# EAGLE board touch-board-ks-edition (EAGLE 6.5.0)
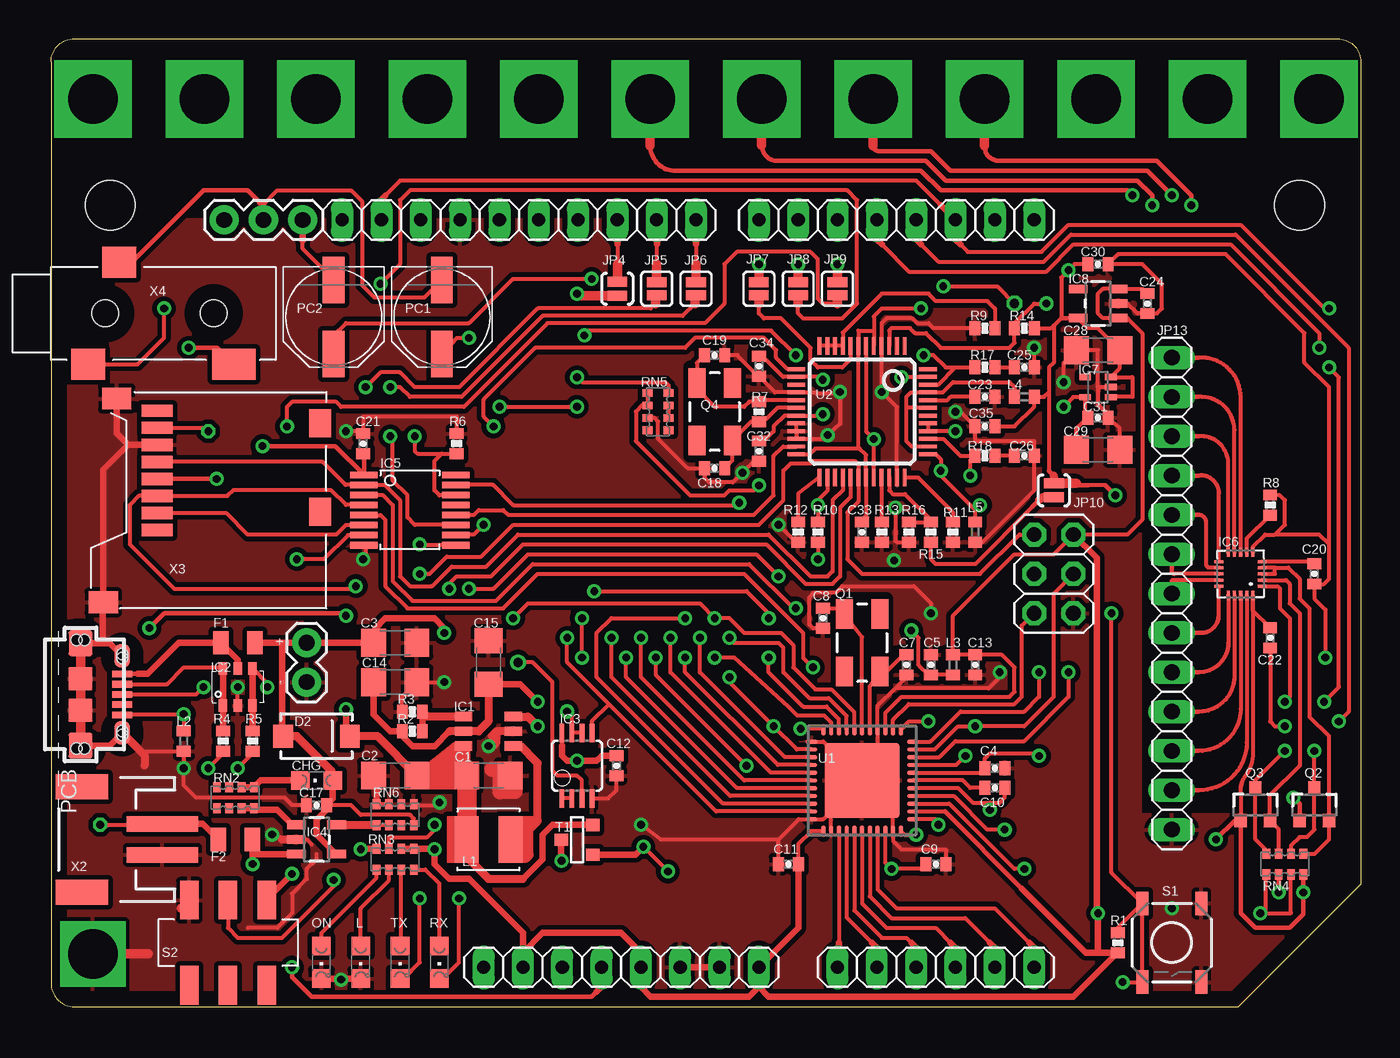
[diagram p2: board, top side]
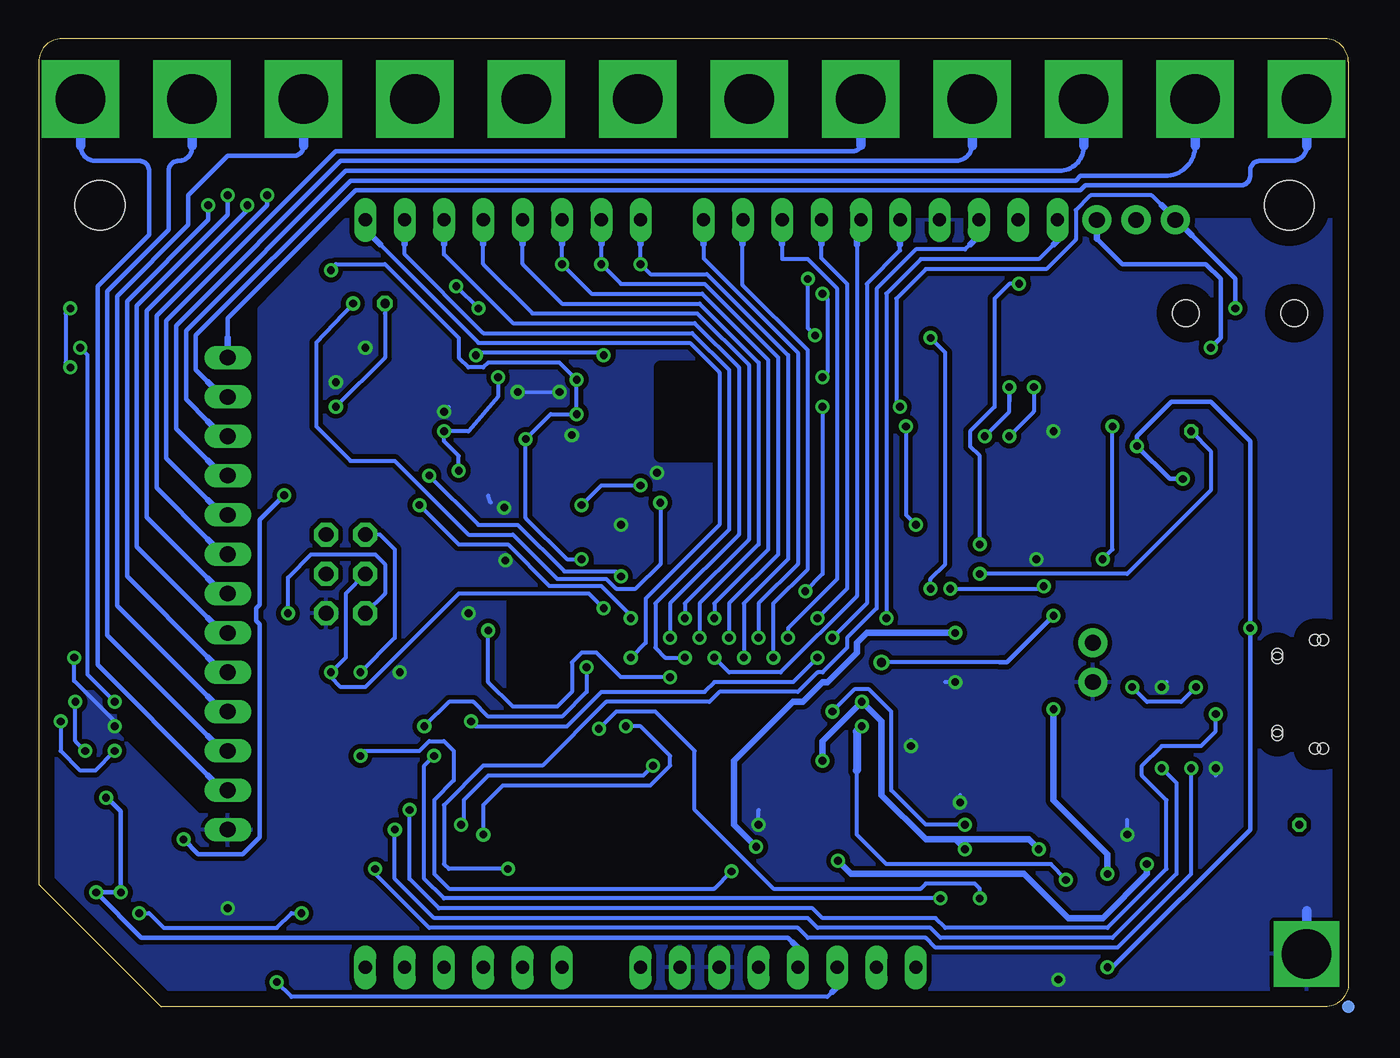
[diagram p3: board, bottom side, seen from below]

Size 84.6 x 62.5 mm. Coordinates in mm from the lower left corner, seen from the top.
Outline: 0,61 0,1.5 arc90 1.5,0 76.7,0 84.6,7.9 84.6,61 arc90 83.1,62.5 1.5,62.5 arc90 0,61
Copper layers (1*16): Top 0.035mm / dielectric 1.5mm / Bottom 0.035mm
Design rules "default *": minimum track width 10mil, minimum drill 20mil, track to track 8mil, track to pad 8mil, pad to pad 8mil, via to via 8mil, smd to smd 8mil, copper to edge 40mil, drill to drill 8mil, minimum pad ring 10mil, minimum via ring 8mil, stop-mask expansion 1.25mil, vias tented up to drill 0mil, thermal gap 10mil
Net classes: 1 power: width 0.254 mm, drill 0.61 mm, clearance 0.254 mm; 2 gnd: width 0.254 mm, drill 0.61 mm, clearance 0.254 mm; 3 usbvcc: width 0.254 mm, drill 0.61 mm, clearance 0.254 mm; 4 aref: width 0.254 mm, drill 0.61 mm, clearance 0.254 mm
Holes 3.2 mm at 80.64,51.75 3.81,51.75
tRestrict: area 41.3,35.6 to 44.5,41.3; area 50.8,20.6 to 54,26.4; area 27.6,9.4 to 28.9,12.2
bRestrict: area 41.3,35.6 to 44.5,41.3; area 50.8,20.6 to 54,26.4

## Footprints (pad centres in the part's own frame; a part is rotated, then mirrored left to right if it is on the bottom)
1206 = smd 1.6 x 1.8: 1 -1.4,0; 2 1.4,0
0402-CAP = smd 0.7 x 0.9: 1 -0.65,0; 2 0.65,0
CHIPLED_0805 = smd 1.2 x 1.2: A 0,-1.05; C 0,1.05
SMA-DIODE = smd 1.27 x 1.47: A -2.15,0; C 2.15,0
0805 = smd 1 x 1.5: 1 -1.1,0; 2 1.1,0
6-LEAD-SOT23 = smd 0.6 x 1.1: 1 -0.95,-1.6; 2 0,-1.6; 3 0.95,-1.6; 4 0.95,1.6; 5 0,1.6; 6 -0.95,1.6
SOT457 = smd 0.8 x 0.55: 1 -1.2,0.95; 2 -1.2,0; 3 -1.2,-0.95; 4 1.2,-0.95; 5 1.2,0; 6 1.2,0.95
MSOP08 = smd 0.3 x 1.2: 1 -0.976,-2.113; 2 -0.326,-2.113; 3 0.324,-2.113; 4 0.974,-2.113; 5 0.974,2.112; 6 0.324,2.112; 7 -0.326,2.112; 8 -0.976,2.112
SOT23-5 = smd 0.55 x 1.2: 1 -0.95,-1.3; 2 0,-1.3; 3 0.95,-1.3; 4 0.95,1.3; 5 -0.95,1.3
TSSOP-16 = smd 0.42 x 1.78: 1 -2.275,-2.97; 2 -1.625,-2.97; 3 -0.975,-2.97; 4 -0.325,-2.97; 5 0.325,-2.97; 6 0.975,-2.97; 7 1.625,-2.97; 8 2.275,-2.97; 9 2.275,2.97; 10 1.625,2.97; 11 0.975,2.97; 12 0.325,2.97; 13 -0.325,2.97; 14 -0.975,2.97; 15 -1.625,2.97; 16 -2.275,2.97
QFN-20-0.4MM = smd 0.6 x 0.2: 1 -1.4,0.8; 2 -1.4,0.4; 3 -1.4,0; 4 -1.4,-0.4; 5 -1.4,-0.8; 11 1.4,-0.8; 12 1.4,-0.4; 13 1.4,0; 14 1.4,0.4; 15 1.4,0.8 | smd 0.2 x 0.6: 6 -0.8,-1.4; 7 -0.4,-1.4; 8 0,-1.4; 9 0.4,-1.4; 10 0.8,-1.4; 16 0.8,1.4; 17 0.4,1.4; 18 0,1.4; 19 -0.4,1.4; 20 -0.8,1.4
SC70 = smd 0.4 x 0.75: 1 -0.65,-0.825; 2 0,-0.825; 3 0.65,-0.825; 4 0.65,0.825; 5 -0.65,0.825
2X03 = drill 0.95 pad 1.55 octagon: 1 -2.54,-1.27; 2 -2.54,1.27; 3 0,-1.27; 4 0,1.27; 5 2.54,-1.27; 6 2.54,1.27
1X08 = drill 0.85 pad 1.422 long: 1 -8.89,0; 2 -6.35,0; 3 -3.81,0; 4 -1.27,0; 5 1.27,0; 6 3.81,0; 7 6.35,0; 8 8.89,0
1X06 = drill 0.85 pad 1.422 long: 1 -6.35,0; 2 -3.81,0; 3 -1.27,0; 4 1.27,0; 5 3.81,0; 6 6.35,0
1X02 = drill 1.016 pad 1.88: 1 0,0; 2 2.54,0
1X10 = drill 0.85 pad 1.422 long: 1 -11.43,0; 2 -8.89,0; 3 -6.35,0; 4 -3.81,0; 5 -1.27,0; 6 1.27,0; 7 3.81,0; 8 6.35,0; 9 8.89,0; 10 11.43,0
SJ_2S-NO = smd 0.635 x 1.27: 1 -0.45,0; 2 0.45,0
SJ_2S = smd 0.635 x 1.27: 1 -0.412,0; 2 0.412,0
1X03 = drill 1.016 pad 1.88: 1 0,0; 2 2.54,0; 3 5.08,0
1X13 = drill 1.016 long: 1 -15.24,0; 2 -12.7,0; 3 -10.16,0; 4 -7.62,0; 5 -5.08,0; 6 -2.54,0; 7 0,0; 8 2.54,0; 9 5.08,0; 10 7.62,0; 11 10.16,0; 12 12.7,0; 13 15.24,0
LQH44PN100MP0L = smd 1.55 x 3: 1 -1.425,0; 2 1.425,0
0402 = smd 0.7 x 0.9: 1 -0.65,0; 2 0.65,0
TP-SP = smd 0.8 x 0.8 bottom: X 0,0
PANASONIC_D = smd 3 x 1.4: + 2.4,0; - -2.4,0
CRYSTAL-SMD-5X3 = smd 1.9 x 1.1: 1 -1.85,-1.15; 2 1.85,-1.15; 3 1.85,1.15; 4 -1.85,1.15
SOT23-3 = smd 0.8 x 0.9: 1 -0.95,-1; 2 0.95,-1; 3 0,1.1
0402-RES = smd 0.7 x 0.9: 1 -0.65,0; 2 0.65,0
CAY16 = smd 0.5 x 0.65: 1 -1.2,-0.675; 2 -0.4,-0.675; 3 0.4,-0.675; 4 1.2,-0.675; 5 1.2,0.675; 6 0.4,0.675; 7 -0.4,0.675; 8 -1.2,0.675
TACTILE_SWITCH_SMD@1 = smd 1.524 x 0.762: 1 -2.54,1.905; 2 2.54,1.905; 3 -2.54,-1.905; 4 2.54,-1.905
JS202011SCQN = smd 1.2 x 2.5: 1 -2.5,-2.75; 2 0,-2.75; 3 2.5,-2.75; 4 -2.5,2.75; 5 0,2.75; 6 2.5,2.75
SOT-23 = smd 0.787 x 0.889: 1 0.025,-1.016; 2 -0.94,1.016; 3 0.991,1.016
QFN44ML7X7 = smd 0.75 x 0.275: 1 -3.275,2.5; 2 -3.275,2; 3 -3.275,1.5; 4 -3.275,1; 5 -3.275,0.5; 6 -3.275,0; 7 -3.275,-0.5; 8 -3.275,-1; 9 -3.275,-1.5; 10 -3.275,-2; 11 -3.275,-2.5; 23 3.275,-2.5; 24 3.275,-2; 25 3.275,-1.5; 26 3.275,-1; 27 3.275,-0.5; 28 3.275,0; 29 3.275,0.5; 30 3.275,1; 31 3.275,1.5; 32 3.275,2; 33 3.275,2.5 | smd 0.275 x 0.75: 12 -2.5,-3.275; 13 -2,-3.275; 14 -1.5,-3.275; 15 -1,-3.275; 16 -0.5,-3.275; 17 0,-3.275; 18 0.5,-3.275; 19 1,-3.275; 20 1.5,-3.275; 21 2,-3.275; 22 2.5,-3.275; 34 2.5,3.275; 35 2,3.275; 36 1.5,3.275; 37 1,3.275; 38 0.5,3.275; 39 0,3.275; 40 -0.5,3.275; 41 -1,3.275; 42 -1.5,3.275; 43 -2,3.275; 44 -2.5,3.275 | smd 4.826 x 4.826: EXP 0,0
LQFP-48 = smd 0.254 x 1.143: 1 -2.75,-4.25; 2 -2.25,-4.25; 3 -1.75,-4.25; 4 -1.25,-4.25; 5 -0.75,-4.25; 6 -0.25,-4.25; 7 0.25,-4.25; 8 0.75,-4.25; 9 1.25,-4.25; 10 1.75,-4.25; 11 2.25,-4.25; 12 2.75,-4.25; 25 2.75,4.25; 26 2.25,4.25; 27 1.75,4.25; 28 1.25,4.25; 29 0.75,4.25; 30 0.25,4.25; 31 -0.25,4.25; 32 -0.75,4.25; 33 -1.25,4.25; 34 -1.75,4.25; 35 -2.25,4.25; 36 -2.75,4.25 | smd 1.143 x 0.254: 13 4.25,-2.75; 14 4.25,-2.25; 15 4.25,-1.75; 16 4.25,-1.25; 17 4.25,-0.75; 18 4.25,-0.25; 19 4.25,0.25; 20 4.25,0.75; 21 4.25,1.25; 22 4.25,1.75; 23 4.25,2.25; 24 4.25,2.75; 37 -4.25,2.75; 38 -4.25,2.25; 39 -4.25,1.75; 40 -4.25,1.25; 41 -4.25,0.75; 42 -4.25,0.25; 43 -4.25,-0.25; 44 -4.25,-0.75; 45 -4.25,-1.25; 46 -4.25,-1.75; 47 -4.25,-2.25; 48 -4.25,-2.75
EDGE-ELEC-LEFT = drill 3.2 pad 5 square: 1 0,0
EDGE-ELEC-RIGHT = drill 3.2 pad 5 square: 1 0,0
EDGE-GND = drill 3.2 pad 4 square: P$1 0,0
EDGE-ELEC = drill 3.2 pad 5 square: 1 0,0
CON2_USB_MICRO_B_AT = smd 0.406 x 1.346: P1 -1.321,2.692; P2 -0.66,2.692; P3 0,2.692; P4 0.66,2.692; P5 1.321,2.692 | smd 1.651 x 1.549: S1 -3.302,0; S2 3.302,0 | smd 1.524 x 1.016: S3 -2.489,2.692; S4 2.489,2.692 | smd 1.524 x 1.524: S5 -1.016,0; S6 1.016,0 | hole 0.7: -3.505,0.254; -3.505,-0.254; 3.505,0.254; 3.505,-0.254; -2.616,2.692; -2.362,2.692; 2.362,2.692; 2.616,2.692
JST-2-SMD = smd 1 x 4.6: 1 -1,-3.7; 2 1,-3.7 | smd 1.6 x 3.4: NC1 -3.4,1.5; NC2 3.4,1.5
MSDC-PP-02 = smd 0.8 x 2: 1 5.06,10.94; 2 6.16,10.94; 3 7.26,10.94; 4 8.36,10.94; 5 9.46,10.94; 6 10.56,10.94; 7 11.66,10.94; 8 12.76,10.94 | smd 1.8 x 1.4: CD1 6.25,0.4; CD2 11.95,0.4 | smd 1.4 x 1.9: S1 0.4,14.4; S2 13.55,13.54
3POLE-JACK = smd 2.2 x 2: 1 2.4,-3.3; 3 4.4,3.3 | smd 2.8 x 2: 2 11.8,-3.3 | hole 1.7: 3.5,0; 10.5,0

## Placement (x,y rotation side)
C1  10uF  [1206]  28.26,14.92 0 top
C2  10uF  [1206]  22.23,14.92 180 top
C3  10uF  [1206]  22.23,23.5 0 top
C4  0.1uF  [0402-CAP]  60.96,15.4 180 top
C5  1uF  [0402-CAP]  56.83,22.07 270 top
C7  22pF  [0402-CAP]  55.24,22.07 270 top
C8  22pF  [0402-CAP]  49.85,25.08 270 top
C9  0.1uF  [0402-CAP]  57.15,9.21 180 top
C10  1uF  [0402-CAP]  60.96,14.13 180 top
C11  0.1uF  [0402-CAP]  47.62,9.21 0 top
C12  0.1uF  [0402-CAP]  36.51,15.56 90 top
C13  0.1uF  [0402-CAP]  59.69,22.07 90 top
C14  10uF  [1206]  22.23,20.95 0 top
C15  10uF  [1206]  28.26,22.23 90 top
C17  1uF  [0402-CAP]  17.14,13.02 0 top
C18  22pF  [0402-CAP]  42.86,34.77 180 top
C19  22pF  [0402-CAP]  42.86,42.07 0 top
C20  0.1uF  [0402-CAP]  81.6,27.94 90 top
C21  0.1uF  [0402-CAP]  20.16,36.35 270 top
C22  0.1uF  [0402-CAP]  78.74,23.81 90 top
C23  1uF  [0402-CAP]  60.33,39.37 0 top
C24  1uF  [0402-CAP]  70.8,45.4 90 top
C25  0.01uF  [0402-CAP]  62.87,41.27 180 top
C26  0.01uF  [0402-CAP]  62.87,35.56 180 top
C28  10uF  [1206]  67.63,42.39 180 top
C29  10uF  [1206]  67.63,35.96 0 top
C30  0.1uF  [0402-CAP]  67.63,47.94 180 top
C31  0.1uF  [0402-CAP]  67.63,38.02 180 top
C32  0.1uF  [0402-CAP]  45.72,35.88 90 top
C33  0.1uF  [0402-CAP]  52.39,30.64 90 top
C34  0.1uF  [0402-CAP]  45.72,41.35 90 top
C35  0.1uF  [0402-CAP]  60.33,37.47 0 top
CHG  Yellow  [CHIPLED_0805]  17.14,14.61 90 top
D2  B340  [SMA-DIODE]  17.14,17.46 0 top
F1  500mA  [0805]  12.06,23.5 0 top
F2  1.1A  [0805]  11.91,10.79 0 top
IC1  MCP1640  [6-LEAD-SOT23]  28.26,17.78 90 top
IC2  ESD Diode  [SOT457]  12.06,20.64 90 top
IC3  LM358  [MSOP08]  33.97,15.56 0 top
IC4  MCP73831  [SOT23-5]  17.14,10.79 270 top
IC5  74HC4050  [TSSOP-16]  23.18,32.07 270 top
IC6  MPR121  [QFN-20-0.4MM]  76.83,27.94 180 top
IC7  1.8V  [SC70]  67.63,40.01 90 top
IC8  MIC5219  [SOT23-5]  67.63,45.4 90 top
ICSP  ICSP  [2X03]  64.77,27.94 270 top
J1  8x1F-H8.5  [1X08]  36.83,2.54 0 top
J2  6x1F-H8.5  [1X06]  57.15,2.54 0 top
J3  8x1F-H8.5  [1X08]  54.61,50.8 180 top
JP1  External  [1X02]  16.51,20.95 90 top
JP3  10x1F-H8.5  [1X10]  30.23,50.8 180 top
JP4  [SJ_2S-NO]  36.58,46.35 90 top
JP5  [SJ_2S]  39.12,46.35 90 top
JP6  [SJ_2S]  41.66,46.35 90 top
JP7  [SJ_2S]  45.72,46.35 90 top
JP8  [SJ_2S]  48.26,46.35 90 top
JP9  [SJ_2S]  50.8,46.35 90 top
JP10  [SJ_2S-NO]  64.77,33.34 90 top
JP11  External Speaker  [1X03]  11.18,50.8 0 top
JP13  Touch Electrodes  [1X13]  72.39,26.67 270 top
L  Red  [CHIPLED_0805]  20,2.86 180 top
L1  LQH44P  [LQH44PN100MP0L]  28.26,10.79 180 top
L2  Ferrite  [0402]  8.57,17.14 90 top
L3  [0402]  58.26,22.07 270 top
L4  Ferrite  [0402]  62.87,39.37 180 top
L5  Ferrite  [0402]  59.69,30.64 270 top
ON  Green  [CHIPLED_0805]  17.46,2.86 180 top
ORIGIN  TP_SP  [TP-SP]  0,0 0 top
PC1  220uF  [PANASONIC_D]  25.24,44.53 270 top
PC2  220uF  [PANASONIC_D]  18.26,44.53 270 top
Q1  16MHz  [CRYSTAL-SMD-5X3]  52.39,23.5 270 top
Q2  BSS138  [SOT23-3]  81.6,13.02 0 top
Q3  BSS138  [SOT23-3]  77.79,13.02 0 top
Q4  12.288MHz  [CRYSTAL-SMD-5X3]  42.86,38.42 270 top
R1  75k  [0402-RES]  68.9,4.13 90 top
R2  976K  [0402-RES]  23.34,17.78 180 top
R3  309K  [0402-RES]  23.34,19.05 180 top
R4  22R  [0402-RES]  11.11,17.14 270 top
R5  22R  [0402-RES]  13.02,17.14 270 top
R6  75k  [0402-RES]  26.19,36.35 90 top
R7  976k  [0402-RES]  45.72,38.42 90 top
R8  75k  [0402-RES]  78.74,32.38 90 top
R9  75k  [0402-RES]  60.33,43.81 180 top
R10  75k  [0402-RES]  48.26,30.64 270 top
R11  75k  [0402-RES]  58.26,30.64 270 top
R12  75k  [0402-RES]  49.53,30.64 90 top
R13  75k  [0402-RES]  53.66,30.64 270 top
R14  75k  [0402-RES]  62.87,43.81 180 top
R15  75k  [0402-RES]  55.4,30.64 270 top
R16  75k  [0402-RES]  56.83,30.64 90 top
R17  22R  [0402-RES]  60.33,41.27 0 top
R18  22R  [0402-RES]  60.33,35.56 0 top
RN2  1K  [CAY16]  11.91,13.49 180 top
RN3  1K  [CAY16]  22.23,9.53 180 top
RN4  1K  [CAY16]  79.69,9.21 180 top
RN5  10k  [CAY16]  39.21,38.42 270 top
RN6  10K  [CAY16]  22.23,12.38 0 top
RX  Yellow  [CHIPLED_0805]  25.08,2.86 180 top
S1  RESET  [TACTILE_SWITCH_SMD@1]  72.39,4.13 270 top
S2  DPDT  [JS202011SCQN]  11.43,4.13 0 top
T1  FDN340P  [SOT-23]  33.97,10.79 270 top
TX  Yellow  [CHIPLED_0805]  22.54,2.86 180 top
U1  ATMEGA32U4  [QFN44ML7X7]  52.39,14.61 180 top
U2  VS1053  [LQFP-48]  52.39,38.42 180 top
U$1  EDGE-ELEC-LEFT  [EDGE-ELEC-LEFT]  2.7,58.6 0 top
U$3  EDGE-ELEC-RIGHT  [EDGE-ELEC-RIGHT]  81.9,58.6 0 top
U$6  EDGE-GND  [EDGE-GND]  2.7,3.4 0 top
U$8  OSHW-LOGO  [OSHW-LOGO]  not placed on the board
U$17  EDGE-ELEC  [EDGE-ELEC]  74.7,58.6 0 top
U$18  EDGE-ELEC  [EDGE-ELEC]  67.5,58.6 0 top
U$22  EDGE-ELEC  [EDGE-ELEC]  60.3,58.6 0 top
U$24  EDGE-ELEC  [EDGE-ELEC]  53.1,58.6 0 top
U$26  EDGE-ELEC  [EDGE-ELEC]  45.9,58.6 0 top
U$27  EDGE-ELEC  [EDGE-ELEC]  38.7,58.6 0 top
U$28  EDGE-ELEC  [EDGE-ELEC]  31.5,58.6 0 top
U$29  EDGE-ELEC  [EDGE-ELEC]  24.3,58.6 0 top
U$30  EDGE-ELEC  [EDGE-ELEC]  17.1,58.6 0 top
U$31  EDGE-ELEC  [EDGE-ELEC]  9.9,58.6 0 top
X1  USB MICRO  [CON2_USB_MICRO_B_AT]  1.91,20.16 270 top
X2  Batt  [JST-2-SMD]  3.49,10.79 90 top
X3  MICRO-SD  [MSDC-PP-02]  17.78,25.72 90 top
X4  [3POLE-JACK]  0,44.77 0 top

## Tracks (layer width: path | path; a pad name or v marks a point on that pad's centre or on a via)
1.8V  (via drill 0.5, 0.6)
  Top 0.254: C29.1 66.23,37.35 C31.2 66.8,38.27 IC7.5 66.03,39.35 v65.41,38.73 | U2.24 49,35.67 49.37,36.04 52.23,36.04 | C33.2 52.39,31.43 52.64,31.68 U2.31 52.64,35.63 52.23,36.04 | v56.2,45.09 53.66,45.09 53.14,44.56 U2.5 53.14,43.66 52.14,43.66 U2.7 52.14,36.13 52.23,36.04 | v57.63,46.51 61.12,46.51 v62.23,45.4
  Bottom 0.254: v57.63,46.51 v56.2,45.09 | v65.41,38.73 62.23,41.91 62.23,44.77 v62.23,45.4
3.3V  (via drill 0.5, 0.6)
  Top 0.254: RN4.8 80.96,8.46 | Q3.1 76.83,12.33 | 76.83,12.34 Q3.1 | C22.2 77.64,25.57 IC6.20 77.64,16.36 arc-37 77.15,14.92 arc42 76.83,13.81 76.83,12.34 | U2.6 52.64,37.15 v53.14,36.65 U2.32 | IC7.1 68.47,39.37 69.85,39.37 69.85,40.64 69.83,40.66 IC7.3 69.03,41.23 C28.1 69.03,42.41 67.63,43.81 66.97,43.81 IC8.5 | v49.85,38.26 49.85,38.17 U2.19 47.38,38.17 46.67,37.47 46.67,37.15 46.05,36.53 C32.2 | v49.85,40.48 49.85,40.67 U2.14 47.28,40.67 45.95,42 C34.2 | R12.1 v49.53,28.89 | 76.83,12.34 76.83,12.33 | 20.21,35.66 C21.2 | 65.25,44.45 | 65.25,44.45 IC8.5 | IC8.5 65.25,44.45 | 65.25,44.45 | JP10.2 64.9,33.66 | 64.77,43.97 65.25,44.45 | 65.25,44.45 65.25,47.07 v65.72,47.55 66.12,47.94 C30.2 | 64.77,43.97 64.77,41.59 64.45,41.27 64.45,39.69 | C35.2 62.23,37.47 63.52,38.75 L4.1 64.14,39.37 64.45,39.69 | 76.83,12.33 Q3.1 | R14.1 64.61,43.81 64.77,43.97 | 64.45,39.69 64.45,34.61 | 34.29,14.61 IC3.3 34.3,14.6 34.29,14.61 | 34.29,14.61 33.97,14.92 32.7,14.92 32.38,15.24 32.38,20.95 31.11,22.23 v30.16,22.23 | 68.1,33.66 66.99,33.66
  Top 0.305: X3.4 v10.69,34.08 | RN4.8 v80.89,7.37 80.89,5.96 80.01,5.08 77.79,5.08 76.83,6.03 Q3.1 | 20.21,35.66 IC5.1 18.36,36.2 v13.65,36.2 | Q2.1 80.65,13.09 v80.25,13.49 | Q3.1 76.47,12.02 v75.25,10.79 | 68.1,33.66 v68.74,33.02 | 35.56,1.27 34.92,0.64 16.83,0.64 15.56,1.91 v15.56,2.54 | RN4.6 v79.29,7.37 | 64.77,34.29 64.45,34.61 | 66.22,33.79 66.36,33.66 66.99,33.66 | v6.35,24.45 7.3,25.4 18.89,25.4 v19.05,25.24
  Top 0.406: 35.24,0.95 35.56,1.27 J1.4
  Top 0.508: 64.77,34.29 JP10.2
  Top 0.61: 66.22,33.79 JP10.2
  Bottom 0.254: v49.53,28.89 50.48,28.89 53.14,31.55 v53.14,36.65 51.53,38.26 v49.85,38.26 v49.85,40.48 50.96,41.59 55.56,41.59 55.88,41.27 56.83,41.27 57.47,41.91 57.47,43.18 62.23,47.94 65.41,47.94 65.72,47.62 v65.72,47.55 | 80.17,13.49 v80.25,13.49 | 22.54,22.23 v30.16,22.23
  Bottom 0.305: 35.88,4.13 36.2,4.45 77.97,4.45 v80.89,7.37 v79.29,7.37 79.29,12.62 80.17,13.49 | v10.69,34.08 11.54,34.08 v13.65,36.2 13.65,36.83 11.43,39.05 8.89,39.05 6.35,36.51 v6.35,24.45 6.35,11.43 15.24,2.54 v15.56,2.54 | v75.25,10.79 74.3,9.84 71.44,9.84 70.33,10.95 70.33,24.69 70.56,24.92 70.56,25.72 70.33,25.96 70.33,31.43 v68.74,33.02 | v19.05,25.24 22.07,22.23 22.54,22.23
  Bottom 0.406: 35.88,4.13 35.56,3.81 J1.4
5V  (via drill 0.5)
  Top 0.254: L3.1 58.1,22.54 | L3.1 58.26,25.24 62.23,29.21 64.77,29.21 ICSP.2 69.53,30.48 70.48,31.43 70.48,43.5 69.53,44.45 IC8.1 67.94,44.45 67.63,44.77 67.63,46.04 67.94,46.35 IC8.3 70.5,46.35 C24.2 | C13.2 L3.1 | 78.42,8.46 78.42,8.53 RN4.5 | RN4.5 arc90 78.42,8.46 | RN4.5 arc90 78.42,8.46 | 78.42,8.46 78.42,6.03 | 78.42,6.03 80.09,6.03 RN4.7 | 68.88,3.49 R1.1 | U1.34 49.11,11.33 48.26,10.48 48.26,9.86 C11.2 | U1.2 57.72,12.61 | U1.14 53.89,18.96 54.93,20 61.91,20 62.23,20.32 62.23,21.91 61.42,22.72 C13.2 | 59.7,22.54 C13.2 | 78.42,6.03 v78.11,6.03
  Top 0.305: 57.72,12.61 62.71,7.62 | IC3.8 33,16.85
  Top 0.406: 30.48,3.49 31.75,4.76 36.83,4.76 38.1,3.49 J1.5 38.1,1.27 38.73,0.64 45.09,0.64 45.72,1.27 | 45.72,1.27 J1.8 48.27,5.09 C11.2 | 68.88,3.49 68.88,3.48 66.04,0.64 46.35,0.64 45.72,1.27 | 30.48,3.49 30.48,4.76 26.99,8.26 25.72,8.26 24.77,9.21 v24.77,10.16 24.73,10.2 RN3.1 RN3.2 | 30.48,3.49 J1.2 | R1.1 67.63,3.48 | 67.63,3.48 66.85,3.48 62.71,7.62 | ICSP.2 67.55,28.97 67.55,6.11 v67.63,6.03 67.63,3.48 | 20.64,20.77 C14.1 20.82,18.86 21.91,17.78 R2.2 22.69,17.48 23.34,16.83 24.77,16.83 25.72,17.78 | C12.2 35.58,16.21 35.24,15.88 v33.97,15.88 33.34,15.88 33,16.22 33,16.85 | C15.1 30.29,20.82 v31.43,19.68 | RN3.4 20.04,10.2 v20,10.16
  Top 0.508: 25.72,17.78 IC1.5 27.62,17.78 28.26,18.41 C15.1
  Bottom 0.254: v78.11,6.03 77.47,6.03 76.52,5.08 69.22,5.08 68.26,6.03 v67.63,6.03
  Bottom 0.406: v33.97,15.88 33.97,17.14 v31.43,19.68 30.16,18.41 30.16,13.65 27.3,10.79 25.4,10.79 | v20,10.16 20.64,10.79 25.4,10.79 | 25.4,10.79 v24.77,10.16
A0
  Top 0.254: U1.36 50.89,4.14
  Top 0.406: 50.89,4.14 50.89,2.63 J2.1
A1
  Top 0.254: U1.37 51.39,5.76 53.02,4.13
  Top 0.406: 53.02,4.13 53.34,3.81 J2.2
A2
  Top 0.254: U1.38 51.89,6.21 53.66,4.45 55.24,4.45 55.56,4.13
  Top 0.406: 55.56,4.13 55.88,3.81 J2.3
A3
  Top 0.254: U1.39 52.39,6.67 53.98,5.08 57.15,5.08 58.1,4.13
  Top 0.406: 58.1,4.13 58.42,3.81 J2.4
A4
  Top 0.254: U1.40 52.89,7.12 54.29,5.71 59.05,5.71 60.64,4.13
  Top 0.406: 60.64,4.13 60.96,3.81 J2.5
A5
  Top 0.254: U1.41 53.39,7.57 54.61,6.35 60.96,6.35 63.18,4.13
  Top 0.406: 63.18,4.13 63.5,3.81 J2.6
AGND  (via drill 0.5)
  Top 0.254: U2.37 57.15,35.67 57.47,35.35 v57.47,34.61 57.47,34.29 59.69,32.07 | v54.93,40.64 54.93,40.67 U2.47 | v28.97,38.73 v33.97,38.73 | v46.35,25.08 46.35,25.4 44.93,26.83 v35.08,26.83 | v58.42,37.15 58.42,37.17 U2.40 U2.41 | L5.1 59.69,32.07 | X4.1 5.59,41.47 7.3,43.18 v7.3,45.09 | v60.01,32.38 59.69,32.07
  Bottom 0.254: v54.93,40.64 54.93,39.37 56.83,37.15 v58.42,37.15 58.42,36.51 57.47,35.56 v57.47,34.61 | v33.97,38.73 33.97,27.94 v35.08,26.83 | v46.35,25.08 46.35,25.24 48.26,27.15 51.59,27.15 54.29,29.84 57.47,29.84 v60.01,32.38 | v28.97,38.73 29.21,38.97 29.21,45.72 27.3,47.62 19.53,47.62 17.62,49.53 17.62,51.44 16.67,52.39 12.7,52.39 12.06,51.75
  Bottom 0.305: v7.3,45.09 7.3,46.99 10.16,49.85
  Bottom 0.406: 12.06,51.75 11.18,50.86 JP11.1 11.11,50.8 10.16,49.85
AREF  (via drill 0.5)
  Top 0.254: U1.42 53.89,9.29 v54.29,8.89 56.18,8.89 C9.2
  Bottom 0.254: 24.43,49.23 24.77,48.9 27.94,48.9 30.48,46.35 30.48,25.72 32.38,23.81 32.38,23.18 33.97,21.59 34.29,21.59 35.56,20.32 40.64,20.32 41.27,19.68 47.94,19.68 52.07,15.56 55.88,15.56 58.42,13.02 58.42,9.21 58.1,8.89 v54.29,8.89
  Bottom 0.406: JP3.8 23.88,49.78 24.43,49.23
AVCC  (via drill 0.5)
  Top 0.254: U1.24 48.16,16.61 v46.67,18.1 43.81,20.95 v43.81,21.27 | L3.2 C5.2 56.67,21.42 56.04,22.05 56.04,23.81 v55.56,24.29 | U1.44 55.1,11.11 v55.88,11.11
  Bottom 0.254: v46.67,18.1 45.72,18.1 43.81,16.19 43.81,15.56 45.09,14.29 54.61,14.29 55.88,13.02 v55.88,11.11 | v55.56,24.29 55.56,20.95 53.98,19.37 51.12,19.37 50.16,20.32 50.16,22.23 49.53,22.86 48.58,22.86 46.99,21.27 v43.81,21.27
AVDD
  Top 0.254: U2.38 55.59,36.17 55.24,36.51 55.24,38.67 | U2.43 55.24,38.67 | 55.24,38.67 55.24,39.37 55.54,39.67 U2.45 57.61,39.67 58.26,40.32 61.91,40.32 62.22,40.02 L4.2 62.23,39.7
D0/RX  (via drill 0.5)
  Top 0.254: v46.35,22.54 46.35,21.59 48.58,19.37 50.09,19.37 50.89,18.57 U1.20
  Bottom 0.254: v46.35,22.54 45.4,23.5 45.4,26.35 40.64,31.11 40.64,40.96 42.55,42.86 56.2,42.86 62.55,49.21
  Bottom 0.406: 62.55,49.21 63.5,50.16 J3.1
D1/TX  (via drill 0.5)
  Top 0.254: v42.86,22.54 44.13,22.54 47.62,19.37 48.18,18.81 49.93,18.81 50.39,18.35 U1.21
  Bottom 0.254: v42.86,22.54 44.13,22.54 44.77,23.18 44.77,26.04 40.01,30.8 40.01,41.12 42.39,43.5 55.88,43.5 60.96,48.58 60.96,49.21
  Bottom 0.406: 60.96,49.21 J3.2
D2/SDA  (via drill 0.5)
  Top 0.254: 21.57,52.37 22.54,53.34 55.88,53.34 57.47,51.75 | U1.19 51.39,18.78 50.24,19.92 48.97,19.92 47.31,21.59 47.31,23.18 46.99,23.5 44.13,23.5 v43.81,23.81 | 81.6,13.97 v81.6,16.51 Q2.3 81.6,11.43 81.12,10.95 80.64,10.95 80.09,10.4 RN4.2 | 82.55,19.68 v82.23,19.68 83.19,20.64 83.19,40.64 v82.55,41.27 82.87,40.96 | v82.55,45.09 82.23,45.09 76.83,50.48 65.72,50.48 63.98,48.74 59.21,48.74 58.74,49.21
  Top 0.406: 21.57,52.37 21.34,52.13 JP3.9 | 58.74,49.21 58.42,49.53 J3.3 57.47,51.75
  Bottom 0.254: v82.23,19.68 82.23,17.14 v81.6,16.51 | v43.81,23.81 43.81,26.04 39.37,30.48 39.37,41.27 42.23,44.13 53.98,44.13 58.42,48.58 58.42,49.21 | v82.55,45.09 82.87,44.77 82.87,41.59 v82.55,41.27
  Bottom 0.406: 58.42,49.21 J3.3
D2/SDA_L
  Top 0.254: RN4.1 80.93,9.84 81.6,9.84 82.55,10.79 Q2.2 82.55,12.34 82.55,17.46 81.28,18.73 81.28,25.72 80.64,26.35 80.64,27.62 79.93,28.34 79.06,28.34 | 79.06,28.34 IC6.4 | IC6.3 79.06,27.94 79.06,28.34
D3/SCL  (via drill 0.5)
  Top 0.254: U1.18 51.89,18.99 50.4,20.48 49.37,20.48 47.94,21.91 47.94,23.34 47.15,24.13 44.77,24.13 43.81,25.08 v42.86,25.08 41.91,26.04 30.8,26.04 v29.84,25.08 | RN4.4 78.42,9.95 78.42,10.16 77.79,10.79 Q3.3 77.79,14.61 v79.69,16.51 | v83.19,18.41 83.82,19.05 83.82,42.55 76.52,49.85 65.88,49.85 64.14,48.1 57.31,48.1 56.2,49.21
  Top 0.406: 56.2,49.21 55.88,49.53 J3.4
  Bottom 0.254: 19.03,49.23 20,48.26 27.62,48.26 29.84,46.04 v29.84,25.08 | v42.86,25.08 42.86,26.04 38.73,30.16 38.73,41.43 42.07,44.77 52.7,44.77 55.88,47.94 55.88,49.21 | v83.19,18.41 83.19,16.51 81.92,15.24 80.96,15.24 v79.69,16.51
  Bottom 0.406: JP3.10 18.8,49.47 19.03,49.23 | 55.88,49.21 J3.4
D3/SCL_L
  Top 0.254: RN4.3 79.29,11.46 Q3.2 78.74,13.65 80.64,15.56 80.64,25.4 80.01,26.04 80.01,27.3 79.78,27.54 IC6.2
D4/IRQ  (via drill 0.5)
  Top 0.254: 48.35,16.11 U1.25 47.4,16.11 41.91,21.59 v41.91,23.81 | IC6.1 79.22,27.14 79.38,26.99 79.38,25.72 80.01,25.08 80.01,20 v79.69,19.68 | 53.66,49.21 55.4,47.47 64.29,47.47 66.04,49.21 76.2,49.21 81.92,43.5 v81.92,42.55
  Top 0.406: 53.66,49.21 53.34,49.53 J3.5
  Bottom 0.254: v81.92,42.55 81.44,42.07 81.44,21.43 v79.69,19.68 | v41.91,23.81 41.91,26.04 38.1,29.84 38.1,41.59 41.91,45.4 50.8,45.4 53.34,47.94 53.34,49.21
  Bottom 0.406: 53.34,49.21 J3.5
D5*/SD-CS  (via drill 0.5)
  Top 0.254: U1.31 43.41,13.11 35.24,21.27 35.24,24.13 36.2,25.08 v40.96,25.08
  Top 0.61: JP9.2 v50.8,47.94
  Bottom 0.254: v40.96,25.08 40.96,26.04 37.47,29.53 37.47,41.75 41.75,46.04 48.9,46.04 v50.8,47.94 50.8,49.21
  Bottom 0.406: 50.8,49.21 J3.6
D5*/SD-CS-*  (via drill 0.5)
  Top 0.254: 50.8,45.4 49.85,45.4 49.53,45.72 49.53,48.26 49.05,48.74 44.29,48.74 43.5,47.94 43.5,45.4 42.23,44.13 32.07,44.13 26.67,38.73 18.73,38.73 18.41,39.05 15.56,39.05 15.24,38.73 v15.24,37.47 | IC5.7 19.17,30.44 17.62,28.89 v15.88,28.89
  Top 0.61: JP9.1 50.8,45.4
  Bottom 0.254: v15.88,28.89 15.24,29.53 v15.24,37.47
D6*/MP3-DCS  (via drill 0.5)
  Top 0.254: U1.27 46.49,15.11 40.01,21.59 v40.01,23.81
  Top 0.61: JP8.2 v48.26,47.94
  Bottom 0.254: v40.01,23.81 40.01,26.04 36.83,29.21 36.83,41.91 41.59,46.67 46.99,46.67 v48.26,47.94 48.26,49.21
  Bottom 0.406: 48.26,49.21 J3.7
D6*/MP3-DCS-*  (via drill 0.5)
  Top 0.254: 48.26,45.4 48.26,44.77 48.58,44.45 51.12,44.45 52.07,45.4 52.07,52.07 51.44,52.7 23.18,52.7 22.54,52.07 22.54,47.94 22.23,47.62 21.91,47.31 v21.27,46.67 | IC5.9 23.86,29.79 v23.81,29.84
  Top 0.61: JP8.1 48.26,45.4
  Bottom 0.254: v23.81,29.84 23.81,35.56 24.45,36.2 24.45,37.15 22.86,38.73 22.86,45.72 21.91,46.67 v21.27,46.67
D7/MP3-DREQ  (via drill 0.5)
  Top 0.254: v39.05,22.54 39.05,21.43 v44.93,15.56 | v57.31,11.75 57.11,12.11 U1.1
  Top 0.61: JP7.2 v45.72,47.94
  Bottom 0.254: v39.05,22.54 39.05,26.04 36.2,28.89 36.2,42.07 41.43,47.31 45.09,47.31 v45.72,47.94 45.72,49.21 | v44.93,15.56 45.56,14.92 55.56,14.92 57.15,13.34 57.15,11.91 v57.31,11.75
  Bottom 0.406: 45.72,49.21 J3.8
D7/MP3-DREQ-*
  Top 0.254: U2.8 51.64,41.8 51.12,41.27 49.53,41.27 49.05,41.75 49.05,42.55 47.15,44.45 46.04,44.45 45.72,44.77 45.72,45.4
  Top 0.61: JP7.1 45.72,45.4
D+  (via drill 0.5)
  Top 0.254: X1.P3 9.37,20.16 v9.84,20.64 | IC2.4 13.97,20.88 v13.97,20.64
  Top 0.406: IC2.3 | R5.1 IC2.3 | IC2.3 IC2.4
  Bottom 0.254: v9.84,20.64 10.79,19.68 13.02,19.68 v13.97,20.64
D-
  Top 0.254: X1.P2 7.49,20.82 8.57,21.91 11.04,21.91 IC2.6
  Top 0.406: IC2.6 IC2.1 R4.1
ELE0
  Top 0.254: IC6.8 76.83,39.37 arc93 74.14,41.91
  Top 0.305: 74.14,41.91 JP13.1
  Bottom 0.305: 72.39,43.18 72.39,44.45 64.14,52.7 17.3,52.7 16.99,53.02 6.99,53.02 arc-90 6.35,53.66 6.35,53.98 arc90 5.71,54.61 3.65,54.61 arc-90 2.7,55.56
  Bottom 0.406: 72.39,43.18 JP13.1
  Bottom 0.61: U$1.1 2.7,55.56
ELE1
  Top 0.254: IC6.9 76.44,37.23 arc94 74.14,39.37
  Top 0.305: 74.14,39.37 JP13.2
  Bottom 0.305: 73.66,40.32 74.45,41.12 74.45,43.34 64.45,53.34 17.62,53.34 17.3,53.66 11.83,53.66 arc-90 9.9,55.58
  Bottom 0.406: 73.66,40.32 72.71,39.37 JP13.2
  Bottom 0.61: U$31.1 9.9,55.58
ELE2
  Top 0.254: IC6.10 76.03,35.09 arc95 74.14,36.83
  Top 0.305: 74.14,36.83 JP13.3
  Bottom 0.305: 73.66,37.78 75.09,39.21 75.09,43.66 64.77,53.98 18.66,53.98 arc-92 17.1,55.59
  Bottom 0.406: 73.66,37.78 72.71,36.83 JP13.3
  Bottom 0.61: U$30.1 17.1,55.59
ELE3
  Top 0.254: IC6.11 75.44,33.15 arc97 74.14,34.29
  Top 0.305: 74.14,34.29 JP13.4
  Bottom 0.305: 73.66,35.24 75.72,37.31 75.72,43.97 65.09,54.61 25.38,54.61 arc-84 24.3,55.59
  Bottom 0.406: 73.66,35.24 72.71,34.29 JP13.4
  Bottom 0.61: U$29.1 24.3,55.59
ELE4
  Top 0.254: IC6.12 74.85,28.34 arc-90 74.61,28.57 74.61,31.27 arc90 74.14,31.75
  Top 0.305: 74.14,31.75 JP13.5
  Bottom 0.305: 73.66,32.7 76.36,35.4 76.36,44.29 65.41,55.24 31.96,55.24 arc-76 31.5,55.61
  Bottom 0.406: 73.66,32.7 72.71,31.75 JP13.5
  Bottom 0.61: U$28.1 31.5,55.61
ELE5  (via drill 0.5)
  Top 0.254: IC6.13 72.55,27.94 arc-90 72.39,28.1 72.39,28.26
  Top 0.305: v69.85,52.39 69.53,52.7 57.47,52.7 56.2,53.98 40.32,53.98 arc-90 38.7,55.6 | JP13.6 72.39,28.26
  Top 0.61: U$27.1 38.7,55.6
  Bottom 0.305: v69.85,52.39 69.85,51.75 76.99,44.61 76.99,33.5 73.66,30.16
  Bottom 0.406: 73.66,30.16 72.71,29.21 JP13.6
ELE6  (via drill 0.5)
  Top 0.254: IC6.14 72.47,27.54 arc90 72.39,27.46
  Top 0.305: v71.12,51.75 71.12,52.39 70.17,53.34 57.78,53.34 56.52,54.61 46.91,54.61 arc-90 45.9,55.62 | 72.39,27.46 JP13.7
  Top 0.61: U$26.1 45.9,55.62
  Bottom 0.305: v71.12,51.75 71.12,51.44 77.63,44.93 77.63,31.59 73.66,27.62
  Bottom 0.406: 73.66,27.62 72.71,26.67 JP13.7
ELE7  (via drill 0.5)
  Top 0.254: IC6.15 75.4,27.14 75.4,25.23 arc-90 74.3,24.13
  Top 0.305: v72.39,52.39 70.8,53.98 58.1,53.98 56.83,55.24 53.45,55.24 arc-90 53.1,55.6 | JP13.8 74.3,24.13
  Top 0.61: U$24.1 53.1,55.6
  Bottom 0.305: v72.39,52.39 72.39,51.12 78.26,45.24 78.26,29.69 73.66,25.08
  Bottom 0.406: 73.66,25.08 72.71,24.13 JP13.8
ELE8  (via drill 0.5)
  Top 0.254: IC6.16 76.03,23.49 arc-90 74.14,21.59
  Top 0.305: v73.66,51.75 73.66,52.39 71.44,54.61 61.24,54.61 arc-90 60.3,55.55 60.3,55.58 | JP13.9 74.14,21.59
  Top 0.61: U$22.1 60.3,55.58
  Bottom 0.305: v73.66,51.75 73.66,50.8 78.9,45.56 78.9,27.78 73.66,22.54
  Bottom 0.406: 73.66,22.54 72.71,21.59 JP13.9
ELE9
  Top 0.254: IC6.17 76.44,21.35 arc-90 74.14,19.05
  Top 0.305: JP13.10 74.14,19.05
  Bottom 0.305: 73.66,20 79.53,25.88 79.53,45.88 74.93,50.48 74.93,52.39 72.39,54.93 68.14,54.93 arc-92 67.5,55.6
  Bottom 0.406: 73.66,20 72.71,19.05 JP13.10
  Bottom 0.61: U$18.1 67.5,55.6
ELE10
  Top 0.254: IC6.18 76.83,19.21 arc-90 74.14,16.51
  Top 0.305: JP13.11 74.14,16.51
  Bottom 0.305: 73.66,17.46 80.17,23.97 80.17,46.2 76.2,50.16 76.2,53.98 arc90 75.56,54.61 arc-90 74.7,55.48 74.7,55.59
  Bottom 0.406: 73.66,17.46 72.71,16.51 JP13.11
  Bottom 0.61: U$17.1 74.7,55.59
ELE11
  Top 0.254: IC6.19 77.23,17.07 arc-90 74.14,13.97
  Top 0.305: JP13.12 74.14,13.97
  Bottom 0.305: 73.66,14.92 80.8,22.07 80.8,46.51 77.47,49.85 77.47,53.98 arc-90 78.11,54.61 80.93,54.61 arc90 81.9,55.58
  Bottom 0.406: 73.66,14.92 72.71,13.97 JP13.12
  Bottom 0.61: 81.9,55.58 U$3.1
G1
  Top 0.254: U2.12 U2.11 U2.10 U2.9 51.14,43.52 53.66,46.04 56.67,46.04 57.15,45.56 60.48,45.56 60.98,45.07 R9.1
G2
  Top 0.254: U2.25 48.26,33.11 R10.1
GND  (via drill 0.5)
  Top 0.254: U1.35 50.39,12.61 U1.EXP | 52.89,14.11 U1.EXP | U1.EXP 53.39,15.61 U1.15 53.39,19.41 54.53,20.56 | U1.23 49.89,17.11 U1.EXP | U1.EXP 49.89,12.11 U1.33 48.3,12.11 46.98,10.78 | U2.20 U2.21 U2.22 50,36.67 v50.16,36.91 50.96,37.62 v50.96,39.69 | U2.35 54.64,38.71 v53.66,39.69 53.64,39.71 U2.4 53.64,44.11 53.98,44.45 55.64,44.45 55.96,44.13 56.67,44.13 56.99,43.81 R9.2 | C29.2 69.03,37.35 C31.1 68.26,38.1 68.26,38.26 67.63,38.89 67.63,40.01 | 67.63,40.01 67.63,42.39 C28.2 | RN5.3 38.98,38.02 39.21,37.78 39.21,36.67 41.12,34.77 C18.2 42.21,34.15 42.5,33.86 44.04,33.86 v44.67,34.48 45.41,35.23 C32.1 45.7,35.23 | 50.8,39.67 v50.96,39.69 | U1.EXP 54.39,12.61 U1.43 54.39,10.7 54.93,10.16 57.8,10.16 C9.1 | C11.1 46.98,10.78 | IC6.6 77.64,29.69 78.42,30.48 79.06,30.48 | 79.06,30.48 79.69,31.11 79.69,32.7 79.38,33.02 78.75,33.02 R8.2 | 82.55,29.84 81.92,30.48 79.06,30.48 | 82.55,29.84 82.55,27.62 82.22,27.29 C20.1 81.6,26.35 82.31,25.64 v82.31,22.54 | 82.55,29.84 82.55,40.01 80.96,41.59 80.96,43.5 75.88,48.58 68.91,48.58 C30.1 70.48,47.94 71.75,46.67 71.75,45.09 71.44,44.77 70.82,44.77 C24.1 70.79,44.77 70.17,44.77 69.53,45.4 IC8.2 | R6.2 26.19,38.1 20.18,38.1 20.18,37 C21.1 20.02,37.15 v19.05,37.15 | C22.1 78.74,18.41 79.06,18.1 v79.69,18.1 | 46.98,10.78 39.38,10.78 v38.1,11.75 | C28.2 65.72,42.39 | IC7.2 67.63,40.01 | C25.1 63.5,41.59 v63.5,42.55 | C8.2 49.23,24.43 48.97,24.69 48.97,26.43 49.29,26.75 50.72,26.75 51.12,27.15 55.72,27.15 56.83,26.04 v56.83,25.4 | C33.1 52.4,29.84 | L5.2 59.99,29.83 63.52,33.35 C26.1 63.52,36.5 63.5,36.51 59.69,36.51 59.69,37.45 C35.1 58.72,38.42 v58.42,38.42
  Top 0.254: C34.1 45.7,40.64 | v46.99,31.11 48.12,29.99 R10.2 | v50.96,39.69 50.72,39.61 49.37,39.61 49.31,39.67 U2.16 46.75,39.67 C34.1 | 54.53,20.56 60.56,20.56 61.28,21.27 v61.28,21.59 | 54.53,20.56 55.24,21.27 C7.2 | IC5.8 20.32,29.68 20.32,28.89 v20.16,28.89 | 44.35,42.07 C19.2 44.29,42.07 45.66,40.7 C34.1 | v54.53,32.23 54.53,30.08 54.62,29.99 R15.2 | v65.41,40.32 65.41,41.56 C28.2 | RN6.8 RN6.7 21.82,13.25 | 5.77,16.5 L2.1 v8.57,15.4 8.57,14.29 9.37,13.49 15.08,13.49 15.56,13.02 C17.1 | IC3.4 35.99,13.44 36.51,13.97 C12.1 | RN6.5 23.46,13.02 25.08,13.02 v25.08,13.18 | IC2.2 v12.06,20.64 | R3.2 22.69,20.02 C14.2 v25.4,20.95 | 12.7,5.08 14.61,5.08 15.56,6.03 15.56,7.3 16.51,8.26 16.51,8.89 17.14,9.53 17.14,9.84 | 16.19,10.79 15.88,10.79 IC4.2 | v14.29,11.11 14.61,11.11 14.92,10.79 | 16.51,10.79 16.83,10.48
  Top 0.406: 3.33,23.46 3.79,23.46 X1.S3 | X3.6 5,36.28 | X3.S2 4.24,37.03 5,36.28 | 5,36.28 3.38,34.66 X3.S1 3.33,26.07 3.33,23.46 | J1.7 J1.6 | X1.S4 3.79,16.86 X1.S2 | 3.33,23.46 X1.S1 | ON.C L.C | 21.02,14.92 RN6.8 | 28.47,15.32 28.74,15.58
  Top 0.508: IC1.2 29.82,17.82 29.78,17.78 28.78,17.78 28.75,17.75 | 29.06,14.73 29.55,14.73 | 28.47,17.48 28.75,17.75 | 28.75,17.75 28.75,17.04 28.54,16.83 v28.26,16.83 | 14.92,10.79 15.88,10.79 | X1.S4 6.03,16.24 6.03,15.56
  Top 0.61: X1.S2 X1.S6 X1.S5 X1.S1 | U$6.P$1 6.26,3.4 | S2.4 arc-90 8.4,6.35
  Top 1.016: C1.2 29.26,15.32 28.47,15.32 | 28.99,14.8 28.99,13.88 29.01,13.89 29.96,13.89 29.87,13.98 29.3,13.98
  Bottom 0.254: v53.66,39.69 50.82,39.71 arc90 v50.96,39.69 | v50.16,36.91 50.48,36.83 | v56.83,25.4 56.49,25.41 | v38.1,11.75 38.1,12.7 | v72.39,6.35 72.39,6.67 | v46.99,31.11 46.99,31.43 | v65.41,40.32 65.72,40.32 | v58.42,38.42 58.1,38.73 | 55.4,32.54 55.56,33.02 | v79.69,18.1 79.69,18.41 82.31,21.03 v82.31,22.54 | v25.08,13.18 25.08,13.65 | v8.57,15.4 8.57,14.92 | v12.06,20.64 11.75,20.95 | v25.4,20.95 26.04,20.95 | v14.29,11.11 14.29,12.06
  Bottom 0.406: v28.26,16.83 28.26,17.14
  Bottom 0.61: U$6.P$1 2.7,6.19
  other vias: 18.73,1.75 54.45,28.81
  pour Top (isolate 0.305): 0,0 0,50.8 64.77,50.8 70.33,45.09 70.33,12.38 84.77,12.38 84.77,7.94 76.83,0
  pour Bottom (isolate 0.305): 0,0 77.15,0 84.77,7.62 84.77,20.32 79.69,20.32 79.69,17.78 74.3,12.38 70.33,12.38 70.33,45.09 64.77,50.8 0,50.8
GPIO0
  Top 0.254: U2.33 53.64,31.79 R13.1
GPIO1
  Top 0.254: R15.1 R16.2 56.83,31.43 55.17,33.1 54.37,33.1 54.14,33.33 U2.34
IO8/MP3-RST  (via drill 0.5)
  Top 0.254: U1.28 44.77,14.61 38.1,21.27 v38.1,23.81 | 41.67,49.21 41.66,49.2 41.66,47.94
  Top 0.406: JP3.1 41.67,50.78 41.67,49.21
  Top 0.61: JP6.2 41.66,47.94
  Bottom 0.254: v38.1,23.81 38.1,26.04 35.56,28.57 35.56,42.23 41.66,48.32 41.66,49.2 41.67,49.21
  Bottom 0.406: JP3.1 41.67,50.78 41.67,49.21
IO8/MP3-RST-*  (via drill 0.5)
  Top 0.254: 26.17,33.02 IC5.14 26.12,33.02 25.08,33.02 24.77,33.34 24.77,35.24 25.23,35.7 | 25.23,35.7 R6.1 | 41.59,45.4 40.8,44.61 31.75,44.61 26.51,39.37 23.18,39.37 22.54,40.01 v21.91,40.01 | v23.5,36.83 23.5,35.88 23.67,35.7 25.23,35.7
  Top 0.305: JP6.1 41.59,45.88
  Top 0.61: 41.59,45.88 41.59,45.4
  Bottom 0.254: 21.91,39.05 v21.91,40.01 21.91,38.42 v23.5,36.83
IO9*/MP3-CS  (via drill 0.5)
  Top 0.254: U1.29 44.31,14.11 37.15,21.27 v37.15,22.54 | 39.12,46.58 39.12,47.94 39.12,49.2 39.13,49.21
  Top 0.406: JP3.2 39.13,50.78 39.13,49.21
  Top 0.61: 39.12,47.94 JP5.2
  Bottom 0.254: v37.15,22.54 37.15,26.04 34.92,28.26 34.92,42.39 39.13,46.59 39.13,49.21
  Bottom 0.406: JP3.2 39.13,50.78 39.13,49.21
IO9*/MP3-CS-*  (via drill 0.5)
  Top 0.254: IC5.11 26.12,31.11 23.5,31.11 23.02,31.59 23.02,33.02 22.07,33.97 22.07,36.67 v21.91,36.83 | 39.05,45.4 38.73,45.09 31.43,45.09 26.35,40.01 23.5,40.01 22.54,40.96 21.27,40.96 v20.32,40.01
  Top 0.305: JP5.1 39.05,45.88
  Top 0.61: 39.05,45.88 39.05,45.4
  Bottom 0.254: v20.32,40.01 20.32,38.42 v21.91,36.83
IO10*  (via drill 0.5)
  Top 0.254: U1.30 43.86,13.61 36.2,21.27 v36.2,23.81 | 36.59,49.21 36.58,49.2 36.58,47.93
  Top 0.406: JP3.3 36.59,50.78 36.59,49.21
  Top 0.61: JP4.2 36.58,47.93
  Bottom 0.254: v36.2,23.81 36.2,24.45 33.02,27.62 33.02,46.35 34.92,48.26 36.58,48.26 36.58,49.2 36.59,49.21
  Bottom 0.406: JP3.3 36.59,50.78 36.59,49.21
IO11*  (via drill 0.5)
  Top 0.254: v34.29,22.54 v34.29,25.08 | U1.12 55.42,18.41 v56.67,18.41
  Bottom 0.254: v34.29,25.08 32.38,26.99 32.38,46.67 34.05,48.34 34.05,49.21 | v34.29,22.54 35.88,20.95 40.96,20.95 41.59,20.32 48.26,20.32 50.48,18.1 56.36,18.1 v56.67,18.41
  Bottom 0.406: JP3.4 34.05,50.78 34.05,49.21
IO12  (via drill 0.5)
  Top 0.254: U1.26 46.94,15.61 40.96,21.59 v40.96,22.54
  Bottom 0.254: 31.75,49.2 31.75,26.51 36.67,21.59 40.01,21.59 v40.96,22.54
  Bottom 0.406: JP3.5 31.75,50.55 31.75,49.2
IO13*  (via drill 0.5)
  Top 0.254: U1.32 42.96,12.61 36.04,19.53 | IC3.5 34.95,18.45 34.96,18.45 36.04,19.53 | 36.04,19.53 33.34,22.23 v33.34,23.81
  Bottom 0.254: v33.34,23.81 31.11,26.04 31.11,46.67 28.96,48.83 28.96,49.2
  Bottom 0.406: 28.96,49.2 JP3.6
LEFT  (via drill 0.5)
  Top 0.254: 58.42,41.27 R17.1 | v56.36,42.07 56.99,42.07 57.78,41.27 58.42,41.27 | v48.1,42.07 46.51,43.66 34.77,43.66 v34.45,43.34 | v34.92,46.99 29.84,46.99 26.99,44.13 19.05,44.13 18.26,43.34 PC2.+ | U2.46 57.31,40.17 58.42,41.27
  Bottom 0.254: v34.45,43.34 34.92,43.81 v34.92,46.99 | v48.1,42.07 48.26,42.23 56.2,42.23 v56.36,42.07
MIDI-RX  (via drill 0.5)
  Top 0.254: RN5.1 RN5.2 38.18,38.82 37.78,38.42 37.78,36.51 41.27,33.02 43.5,33.02 43.81,33.34 45.4,33.34 v45.72,33.66 | U2.26 50.14,33.31 49.53,32.7 v49.53,32.38 R12.2
  Bottom 0.254: v45.72,33.66 48.26,33.66 v49.53,32.38
MISO  (via drill 0.5)
  Top 0.254: v63.82,21.59 63.82,20 62.87,19.05 58.74,19.05 56.79,17.11 U1.11 | v23.81,27.94 24.45,27.94 25.56,29.05 27.78,29.05 29.84,31.11 45.72,31.11 47.31,32.7 47.31,34.61 47.78,35.08 49.05,35.08 49.21,35.24 51.91,35.24 52.14,35.02 U2.30 52.14,32.61 51.44,31.91 51.44,28.89 52.39,27.94 60.01,27.94 62.55,30.48 ICSP.1 | X3.7 9.93,37.38 v10.16,37.15
  Bottom 0.254: ICSP.1 62.55,30.48 61.59,29.53 61.59,23.81 v63.82,21.59 | v23.81,27.94 14.29,27.94 8.89,33.34 8.89,35.88 v10.16,37.15
MOSI  (via drill 0.5)
  Top 0.254: ICSP.4 64.77,26.67 64.77,20 62.87,18.1 v59.69,18.1 58.58,18.1 57.09,16.61 U1.10 | IC5.5 21.28,31.74 21.59,31.43 21.59,27.15 23.02,25.72 29.21,25.72 31.43,27.94 44.77,27.94 48.58,24.13 48.58,22.54 v49.21,21.91
  Bottom 0.254: v59.69,18.1 58.1,19.68 56.52,19.68 55.56,18.73 50.8,18.73 49.21,20.32 v49.21,21.91
MOSI_L  (via drill 0.5)
  Top 0.254: IC5.4 19.04,32.39 18.1,33.34 11.75,33.34 11.39,32.98 X3.3 5.67,32.98 5.08,32.38 5.08,29.84 7.94,26.99 19.53,26.99 v19.68,27.15 | v25.72,26.99 25.72,27.3 26.19,27.78 28.42,27.78 30.48,29.84 46.2,29.84 48.74,27.3 50.48,27.3 50.96,27.78 50.96,32.23 51.64,32.91 U2.29
  Bottom 0.254: v25.72,26.99 19.84,26.99 v19.68,27.15
MP3-CS_L
  Top 0.254: IC5.12 27.3,31.74 27.62,32.07 29.21,32.07 29.53,31.75 45.4,31.75 46.67,33.02 46.67,35.56 47.28,36.17 U2.23
MP3-DCS_L  (via drill 0.5)
  Top 0.254: U2.13 47.57,41.17 46.83,41.91 46.83,42.39 46.04,43.18 41.59,43.18 40.96,42.55 31.27,42.55 27.94,39.21 27.94,38.1 v28.57,37.47 | IC5.10 26.18,30.48 27.3,30.48 v27.94,31.11
  Bottom 0.254: v28.57,37.47 28.57,31.75 v27.94,31.11
MP3-RST_L  (via drill 0.5)
  Top 0.254: U2.3 54.14,43.66 54.29,43.81 55.48,43.81 55.8,43.5 56.52,43.5 57.47,42.55 61.91,42.55 62.23,42.86 R14.2 62.22,44.12 63.5,45.4 v64.29,45.4 | 26.18,33.66 IC5.15 28.54,33.69 29.84,32.38 44.29,32.38 v44.45,32.54
  Bottom 0.254: v44.45,32.54 44.45,28.57 46.04,26.99 47.31,26.99 47.94,27.62 51.12,27.62 53.98,30.48 56.83,30.48 61.59,35.24 64.45,35.24 66.67,37.47 66.67,42.86 v64.29,45.4
N$1  (via drill 0.5)
  Top 0.254: IC3.6 IC3.7 33.65,18.74 v33.33,19.06 | RN3.3 21.82,10.95 24.29,10.95 24.77,11.43 v24.77,11.75
  Bottom 0.254: v24.77,11.75 27.3,11.75 29.53,13.97 29.53,19.05 30.96,20.48 31.91,20.48 v33.33,19.06
N$2
  Top 0.254: L.A 20,6.35 21.82,8.17 RN3.6
N$3
  Top 0.254: 22.54,8.77 RN3.7 22.62,3.99 TX.A
N$4
  Top 0.406: RN2.7 RN2.8 13.22,12.7 14.61,12.7 15.53,11.78 IC4.1
N$5
  Top 0.254: C23.1 58.1,39.37 57.9,39.17 U2.44
N$6
  Top 0.254: RN3.8 24.17,8.85 25.08,7.94 RX.A
N$8
  Top 0.254: ON.A 17.46,4.76 21.02,8.32 RN3.5
N$9
  Top 0.254: C18.1 44.01,35.27 Q4.3 45.21,37.77 R7.1 46.02,37.77 46.92,38.67 U2.18
N$10
  Top 0.254: C19.1 41.71,41.57 Q4.1 41.71,39.88 42.86,38.73 44.77,38.73 45.1,39.07 R7.2 45.82,39.17 U2.17
N$11
  Top 0.508: L1.1 29.68,9.55 30.68,9.55 30.91,9.78 30.91,11.46 31.32,11.86 | 31.32,11.86 31.14,12.04 30.48,12.04 30.53,11.99 30.53,9.78 30.76,10.01 30.76,11.79 | 31.32,11.86 31.43,11.98 31.43,15.72 30.32,16.83 IC1.1
N$12
  Top 0.406: R3.1 R2.1
  Top 0.508: IC1.4 24.31,18.73 R3.1
N$13  (via drill 0.5)
  Top 0.254: 6.99,11.75 7.14,11.75 X2.2 7.19,11.75 v3.17,11.75
  Top 0.406: F2.1 9.81,11.79 X2.2
N$14  (via drill 0.5)
  Top 0.254: 34.16,45.91 v33.97,46.04 | v33.97,40.64 34.29,40.32 39.69,40.32 39.89,40.12 RN5.8
  Top 0.61: JP4.1 34.1,45.91 arc-90 v33.97,46.04
  Bottom 0.254: v33.97,46.04 33.66,45.72 33.66,40.96 v33.97,40.64
N$15
  Top 0.254: IC3.2 IC3.1
N$19
  Top 0.254: RN6.2 RN6.1 20.98,11.75 20.98,11.74
  Top 0.508: IC4.5 20.99,11.74 arc-90 RN6.1
N$21
  Top 0.254: R17.2 C25.2
N$22
  Top 0.254: C26.2 R18.2
N$23  (via drill 0.5)
  Top 0.254: S2.5 11.43,5.08 12.06,4.45 14.92,4.45 18.26,7.78 v18.26,8.18
  Top 0.508: IC1.3 30.8,18.73 v31.43,18.1
  Bottom 0.254: 31.75,15.24 31.75,11.11 29.84,9.21 19.21,9.21 v18.26,8.18
  Bottom 0.508: v31.43,18.1 31.75,17.78 31.75,15.24
N$24  (via drill 0.5)
  Top 0.254: PC2.- 16.26,48.93 16.26,49.47
  Top 0.305: v8.89,42.55 10.72,42.55 X4.2
  Top 0.406: 16.26,49.47 JP11.3
  Bottom 0.305: 16.26,49.59 14.61,47.94 9.21,47.94 8.26,46.99 8.26,43.18 v8.89,42.55
  Bottom 0.406: 16.26,49.59 JP11.3
N$25
  Top 0.254: 63.37,32.25 59.69,28.57 57.15,28.57 56.83,28.89 R16.1
  Top 0.305: 63.82,32.7 63.37,32.25
  Top 0.508: JP10.1 64,32.89 63.82,32.7
N$26
  Top 0.254: 13.72,51.82 14.61,52.7 19.37,52.7 20.08,51.99 20.08,46.59 20.88,45.8 24.11,45.8 PC1.-
  Top 0.305: X4.3 5.07,48.26 5.4,48.26 9.84,52.7 12.7,52.7 13.49,51.91 13.59,51.82 13.72,51.82
  Top 0.406: JP11.2 13.72,51.69 13.49,51.91
N$27
  Top 0.254: RN5.7 RN5.6
N$32
  Top 0.406: RN2.2 RN2.1 13.54,14.61 CHG.C
N$73
  Top 0.254: U2.36 56,34.17 58.26,31.91 R11.1
RD+  (via drill 0.5)
  Top 0.254: U1.4 58.31,13.61 60.48,11.43 v61.59,11.43 | R5.2 13.02,16.35 v12.06,15.4
  Bottom 0.254: v61.59,11.43 61.59,8.26 59.05,5.71 34.92,5.71 34.29,5.08 26.99,5.08 26.35,4.45 15.24,4.45 11.11,8.57 11.11,14.45 v12.06,15.4
RD-  (via drill 0.5)
  Top 0.254: U1.3 58.02,13.11 62.23,8.89 v62.87,8.89 | R4.2 11.11,16.35 v10.16,15.4
  Bottom 0.254: v62.87,8.89 62.87,8.57 59.37,5.08 35.56,5.08 34.92,4.45 27.3,4.45 26.67,3.81 14.92,3.81 10.16,8.57 v10.16,15.4
RESET  (via drill 0.5)
  Top 0.254: S1.3 68.9,5.08 R1.2 | S1.3 S1.4 v69.22,1.59 | ICSP.5 62.71,24.61 62.71,20 62.23,19.53 55.4,19.53 54.39,18.51 U1.13 | v68.5,25.4 68.5,8.65 S1.3
  Bottom 0.254: v68.5,25.4 68.5,27.7 66.99,29.21 62.87,29.21 62.23,28.57 62.23,26.67 ICSP.5 | 33.34,0.95 33.66,0.64 68.26,0.64 v69.22,1.59
  Bottom 0.406: 33.34,0.95 33.02,1.27 J1.3
REXT
  Top 0.254: IC6.7 77.23,30.23 R8.1
RIGHT  (via drill 0.5)
  Top 0.254: v26.99,26.99 28.57,26.99 30.8,29.21 45.56,29.21 v46.99,27.78 | U2.39 57.63,36.67 58.74,35.56 R18.1 | PC1.+ 26.21,43.18 v26.99,43.18 | 59.67,35.53 R18.1 | v59.37,34.29 59.37,35.26 R18.1
  Bottom 0.254: v26.99,26.99 26.99,27.62 26.04,28.57 26.04,42.23 v26.99,43.18 | 47.15,27.94 v46.99,27.78 47.31,28.1 50.64,28.1 53.66,31.11 56.2,31.11 v59.37,34.29
RXLED  (via drill 0.5)
  Top 0.254: RX.C 25.3,1.81 26.35,2.86 v26.35,6.99 | U1.8 58.47,15.61 v59.05,16.19
  Bottom 0.254: v26.35,6.99 58.42,6.99 59.69,8.26 59.69,15.56 v59.05,16.19
SCK  (via drill 0.5)
  Top 0.254: v65.72,21.59 65.72,20 62.87,17.14 58.42,17.14 57.38,16.11 U1.9 | IC5.3 21.41,33.04 22.07,32.38 22.07,27.46 23.34,26.19 28.73,26.19 31.11,28.57 45.09,28.57 47.94,25.72 v48.1,25.72
  Bottom 0.254: ICSP.3 64.77,26.67 64.77,22.54 v65.72,21.59 65.72,21.27 65.09,20.64 63.5,20.64 57.47,26.67 49.05,26.67 v48.1,25.72
SCK_L
  Top 0.254: X3.5 17.53,35.18 19.01,33.69 IC5.2 21.55,33.69 22.54,32.7 22.54,27.78 23.18,27.15 24.61,27.15 25.88,28.42 28.1,28.42 30.16,30.48 46.35,30.48 49.05,27.78 50.16,27.78 50.48,28.1 50.48,32.7 51.14,33.36 U2.28
SD-CS_L
  Top 0.254: X3.2 11.3,31.88 12.7,30.48 18.41,30.48 19.03,31.09 IC5.6
TXLED  (via drill 0.5)
  Top 0.254: TX.C 22.76,1.81 23.81,2.86 v23.81,6.99 | U1.22 49.83,17.94 v48.42,17.94
  Bottom 0.254: v48.42,17.94 47.31,19.05 44.77,19.05 42.23,16.51 42.23,12.7 37.15,7.62 27.62,7.62 27.3,7.94 24.13,7.94 23.81,7.62 v23.81,6.99
UCAP
  Top 0.254: C10.2 59.37,14.13 58.9,14.61 U1.6
UGND  (via drill 0.5)
  Top 0.254: 60.64,13.18 59.53,13.18 58.6,14.11 U1.5 | 60.64,13.18 61.28,13.18 61.61,13.51 C10.1 | v60.64,12.7 60.64,13.18 | 8.56,17.8 L2.2 | L2.2 8.56,17.78 | L2.2 v8.57,18.89 4.65,18.89 X1.P5
  Bottom 0.254: v60.64,12.7 60.64,8.26 58.74,6.35 34.61,6.35 33.97,5.71 26.67,5.71 26.04,5.08 15.56,5.08 11.75,8.89 11.75,13.34 13.34,14.92 13.34,15.56 12.06,16.83 9.54,16.83 L2.2 v8.57,18.89
V_BATT  (via drill 0.5)
  Top 0.406: T1.1 32.96,9.46 v32.97,9.42 | v13.02,9.21 13.02,9.84 | 13.02,9.84 13.02,10.65 F2.2 13.17,10.8 | IC4.3 15.53,9.84 13.02,9.84
  Bottom 0.406: v13.02,9.21 13.02,8.57 15.88,5.71 18.1,5.71 20.95,8.57 32.12,8.57 v32.97,9.42
VCC  (via drill 0.5)
  Top 0.406: IC1.6 26.86,16.63 26.86,15.42 | 26.86,15.42 C1.1 26.83,14.9 | 30.48,8.26 31.75,9.53 31.75,11.11 32.38,11.75 34.98,11.75 T1.2 | v19.05,19.21 19.05,17.22 D2.C | S2.6 13.93,6.95 v15.56,8.57 | C2.1 26.14,16.92 26.16,14.25 26.16,14.22 25.81,14.22 | 24.28,14.22 25.81,14.22 | 25.81,14.22 25.81,14.61 | 25.81,16.41 25.81,14.61 | 25.81,14.61 24.38,14.61 24.38,14.96 25.58,14.96 25.58,15.29 | 25.58,15.29 24.71,15.29 | 24.41,15.29 24.71,15.29 | 24.71,15.29 25.55,16.13 25.55,15.67 25.3,15.42 | 26.86,15.42 25.7,15.42 25.58,15.29
  Top 0.508: 26.83,9.79 L1.2 26.83,9.68 28.26,8.26 30.48,8.26 | D2.C 21.09,17.46 C2.1
  Top 1.27: L1.2 26.86,10.82 C1.1
  Bottom 0.406: v19.05,19.21 19.05,13.34 15.56,9.84 v15.56,8.57
VREG
  Top 0.254: IC6.5 81.45,28.74 C20.2
VUSB  (via drill 0.5)
  Top 0.254: U1.7 60.31,15.11 C4.2 60.31,16.02 60.64,16.35 63.66,16.35 v63.82,16.19 | v39.85,8.73 v38.26,10.32 | C17.2 19.37,13.02 20,12.38 23.18,12.38 23.43,12.13 RN6.4
  Top 0.406: F1.2 14.92,23.5 | 14.92,23.5 JP1.2 C3.1 20.95,23.62 20.95,24.45 21.59,25.08 24.77,25.08 25.4,24.45 v25.4,24.13 | T1.3 37.74,9.8 v38.26,10.32 | CHG.A 18.2,13.42 C17.2 17.8,12.71 17.14,12.06 17.14,11.11 18.41,9.85 IC4.4 | 14.92,23.5 14.92,17.46 D2.A
  Top 0.508: CHG.A 18.1,14.7 18.1,15.24 15.88,17.46 D2.A
  Bottom 0.254: v63.82,16.19 63.5,16.51 60.01,16.51 59.37,17.14 58.42,17.14 57.78,16.51 57.78,14.61 59.05,13.34 59.05,8.57 58.1,7.62 40.96,7.62 v39.85,8.73
  Bottom 0.406: v38.26,10.32 39.69,11.75 39.69,15.88 35.88,19.68 35.24,19.68 33.97,20.95 33.66,20.95 31.75,22.86 31.75,23.5 31.11,24.13 v25.4,24.13
XTAL1
  Top 0.254: U1.17 52.39,23.88 Q1.1 50.85,25.73 C8.1
XTAL2
  Top 0.254: U1.16 52.89,20.68 Q1.3 53.61,21.26 55.07,22.72 C7.1
XUSB
  Top 0.305: X1.P1 5.61,21.48
  Top 0.406: 5.61,21.48 6.24,21.48 8.26,23.5 F1.1 12.06,22.39 IC2.5
(copper drawn outside any net)
  shapes: Top area x2

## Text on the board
tNames: F1 | + | - | F2
Document: FUSE2 | U$22 | J5 | + | - | U$1 | FUSE | U$3 | + | + | + | + | U$24 | - | - | - | -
